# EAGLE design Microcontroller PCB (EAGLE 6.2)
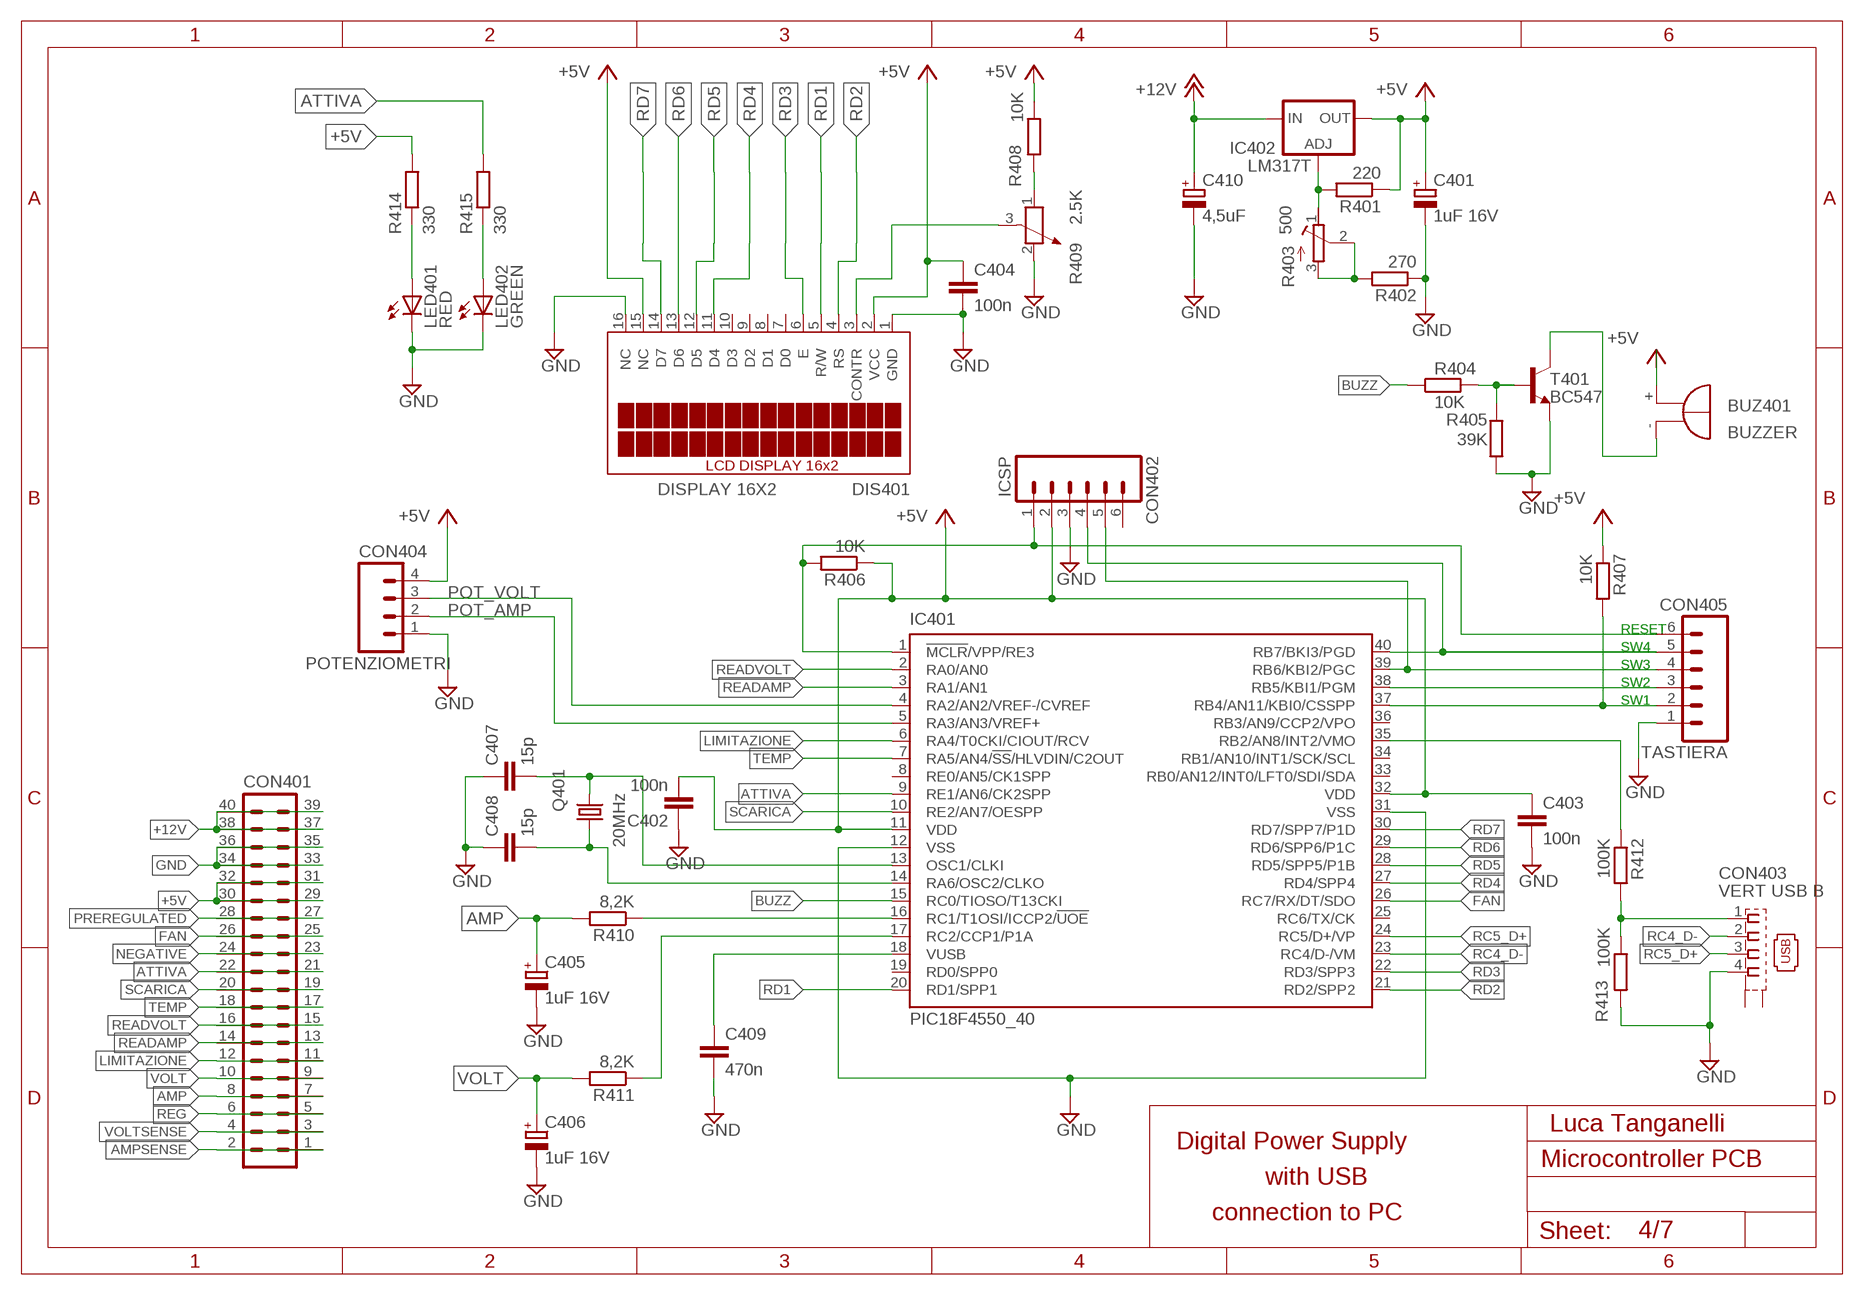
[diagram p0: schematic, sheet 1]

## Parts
BUZ401  BUZZER  F/HMB  [F/HMB]
C401  1uF 16V  CPOL-EUE2.5-5  [E2,5-5]
C402  100n  C-EU025-024X044  [C025-024X044]
C403  100n  C-EU025-024X044  [C025-024X044]
C404  100n  C-EU025-024X044  [C025-024X044]
C405  1uF 16V  CPOL-EUE2.5-5  [E2,5-5]
C406  1uF 16V  CPOL-EUE2.5-5  [E2,5-5]
C407  15p  C-EU025-024X044  [C025-024X044]
C408  15p  C-EU025-024X044  [C025-024X044]
C409  470n  C-EU050-024X044  [C050-024X044]
C410  4,5uF  CPOL-EUE2.5-5  [E2,5-5]
CON401  ML40  [ML40]
CON402  ICSP  MA06  [06PA]
CON403  VERT USB B  KUSBVX-BS1N  [KUSBVX-BS1N]
CON404  POTENZIOMETRI  MA04  [04PA]
CON405  TASTIERA  MA06  [06PA]
DIS401  DISPLAY 16X2  TUXGR_16X2_R2  [TUXGR_16X2_R2]
IC401  PIC18F4550_40  [DIL40]
IC402  LM317T  LM317TS  [317TS]
LED401  RED  LED3MM  [LED3MM]
LED402  GREEN  LED3MM  [LED3MM]
Q401  20MHz  CRYSTALHC49S  [HC49/S]
R401  220  R-EU_0207/10  [0207/10]
R402  270  R-EU_0207/10  [0207/10]
R403  500  R-TRIMMT93YA  [RTRIMT93YA]
R404  10K  R-EU_0207/15  [0207/15]
R405  39K  R-EU_0207/10  [0207/10]
R406  10K  R-EU_0207/22  [0207/22]
R407  10K  R-EU_0207/10  [0207/10]
R408  10K  R-EU_0207/10  [0207/10]
R409  2.5K  POTENTIOMETER_PT-10  [PT-10]
R410  8,2K  R-EU_0207/26  [0207/26]
R411  8,2K  R-EU_0207/26  [0207/26]
R412  100K  R-EU_0207/10  [0207/10]
R413  100K  R-EU_0207/10  [0207/10]
R414  330  R-EU_0207/10  [0207/10]
R415  330  R-EU_0207/22  [0207/22]
T401  BC547  BC547-NPN-TO92-CBE  [TO92-CBE]

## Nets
+5V: BUZ401.+ C401.+ C402.2 C403.1 C404.1 CON401.29 CON401.30 CON401.31 CON401.32 CON402.2 CON404.4 DIS401.2(VCC) DIS401.15(NC) IC401.11(VDD) IC401.32(VDD) IC402.2(OUT) R401.1 R406.1 R407.1 R408.1 R414.2
+12V: C410.+ CON401.37 CON401.38 CON401.39 CON401.40 IC402.3(IN)
AMP: C405.+ CON401.7 CON401.8 R410.2
AMPSENSE: CON401.1 CON401.2
ATTIVA: CON401.21 CON401.22 IC401.9(RE1/AN6/CK2SPP) R415.2
BUZZ: IC401.15(RC0/TIOSO/T13CKI) R404.1
FAN: CON401.25 CON401.26 IC401.26(RC7/RX/DT/SDO)
GND: C401.- C402.1 C403.2 C404.2 C405.- C406.- C407.1 C408.1 C409.2 C410.- CON401.33 CON401.34 CON401.35 CON401.36 CON402.3 CON403.4 CON404.1 CON405.1 DIS401.1(GND) DIS401.16(NC) IC401.12(VSS) IC401.31(VSS) LED401.K(C) LED402.K(C) R402.1 R405.1 R409.2 R413.2 T401.E
LIMITAZIONE: CON401.11 CON401.12 IC401.6(RA4/T0CKI/CIOUT/RCV)
N$1: CON405.3 IC401.38(RB5/KBI1/PGM)
N$2: CON405.2 IC401.37(RB4/AN11/KBI0/CSSPP) R407.2
N$7: IC401.35(RB2/AN8/INT2/VMO) R412.1
N$33: IC402.1(ADJ) R401.2 R403.1(A)
N$34: R402.2 R403.2(S) R403.3(E)
N$35: LED401.A R414.1
N$42: LED402.A R415.1
N$50: CON402.4 CON405.5 IC401.40(RB7/BKI3/PGD)
N$60: CON402.5 CON405.4 IC401.39(RB6/KBI2/PGC)
N$69: IC401.16(RC1/T1OSI/ICCP2/!UOE) R410.1
N$70: IC401.17(RC2/CCP1/P1A) R411.1
N$78: DIS401.3(CONTR) R409.3
N$82: CON403.1 R412.2 R413.1
N$83: C409.1 IC401.18(VUSB)
N$84: C408.2 IC401.14(RA6/OSC2/CLKO) Q401.1
N$85: C407.2 IC401.13(OSC1/CLKI) Q401.2
N$89: R408.2 R409.1
N$91: BUZ401.- T401.C
N$92: R404.2 R405.2 T401.B
NEGATIVE: CON401.23 CON401.24
POT_AMP: CON404.2 IC401.5(RA3/AN3/VREF+)
POT_VOLT: CON404.3 IC401.4(RA2/AN2/VREF-/CVREF)
PREREGULATED: CON401.27 CON401.28
RC4_D-: CON403.2 IC401.23(RC4/D-/VM)
RC5_D+: CON403.3 IC401.24(RC5/D+/VP)
RD1: DIS401.5(R/W) IC401.20(RD1/SPP1)
RD2: DIS401.4(RS) IC401.21(RD2/SPP2)
RD3: DIS401.6(E) IC401.22(RD3/SPP3)
RD4: DIS401.11(D4) IC401.27(RD4/SPP4)
RD5: DIS401.12(D5) IC401.28(RD5/SPP5/P1B)
RD6: DIS401.13(D6) IC401.29(RD6/SPP6/P1C)
RD7: DIS401.14(D7) IC401.30(RD7/SPP7/P1D)
READAMP: CON401.13 CON401.14 IC401.3(RA1/AN1)
READVOLT: CON401.15 CON401.16 IC401.2(RA0/AN0)
REG: CON401.5 CON401.6
RESET: CON402.1 CON405.6 IC401.1(!MCLR!/VPP/RE3) R406.2
SCARICA: CON401.19 CON401.20 IC401.10(RE2/AN7/OESPP)
TEMP: CON401.17 CON401.18 IC401.7(RA5/AN4/!SS!/HLVDIN/C2OUT)
VOLT: C406.+ CON401.9 CON401.10 R411.2
VOLTSENSE: CON401.3 CON401.4
Unconnected: CON402.6 CON403.M1(S1) CON403.M2(S2) DIS401.7(D0) DIS401.8(D1) DIS401.9(D2) DIS401.10(D3) IC401.8(RE0/AN5/CK1SPP) IC401.19(RD0/SPP0) IC401.25(RC6/TX/CK) IC401.33(RB0/AN12/INT0/LFT0/SDI/SDA) IC401.34(RB1/AN10/INT1/SCK/SCL) IC401.36(RB3/AN9/CCP2/VPO)

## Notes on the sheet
- RESET
- SW4
- SW3
- SW2
- SW1
- Luca Tanganelli
- Digital Power Supply
- with USB
- connection to PC
- 4/7

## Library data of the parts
BUZ401 = buzzer:F/HMB: BUZZER; OC_FARNELL: unknown; OC_NEWARK: unknown
C401 C405 C406 C410 = #-rcl:CPOL-EU: POLARIZED CAPACITOR, European symbol
C402-C404 C407-C409 = #-rcl:C-EU: CAPACITOR, European symbol
CON401 = #-con-ml:ML40: HARTING; OC_FARNELL: unknown; OC_NEWARK: unknown
CON402 CON405 = #-con-amp-quick:MA06: AMP QUICK CONNECTOR; OC_FARNELL: unknown; OC_NEWARK: unknown
CON403 = #-con-kycon:KUSBVX-BS1N: USB B-type Receptacle Vertical, 4 Position, Through Hole Source: Sibalco Kycon KUSBVX-BS1N-xxx.pdf
CON404 = #-con-amp-quick:MA04: AMP QUICK CONNECTOR; OC_FARNELL: unknown; OC_NEWARK: unknown
DIS401 = #-display-lcd:TUXGR_16X2_R2: Tuxgraphics LCD display 16x2 characters reflective, without background light Source: tuxgr_12x2_r2.pdf; OC_FARNELL: unknown; OC_NEWARK: unknown
IC401 = #-microchip:PIC18F4*_40: USB Microcontrollers with nanoWatt Technology High-Performance, Enhanced Flash, 28/40/44-Pin, Source: http://ww1.microchip.com/downloads/en/devicedoc/39632c.pdf; MF: MICROCHIP; MPN: PIC18F4550-I/P; OC_FARNELL: 9321357; OC_NEWARK: 74K8623
IC402 = #-v-reg:LM317TS: VOLTAGE REGULATOR
LED401 LED402 = #-led:LED: LED
Q401 = #-crystal:CRYSTAL: CRYSTAL; OC_FARNELL: 1667008; OC_NEWARK: unknown
R401 R402 R404-R408 R410-R415 = #-rcl:R-EU_: RESISTOR, European symbol
R403 = #-rcl:R-TRIMM: Trimm resistor
R409 = #-rcl:POTENTIOMETER_: Potentiometer
T401 = #-transistor:*-NPN-: NPN Transistror BF959 corrected 2008.03.06

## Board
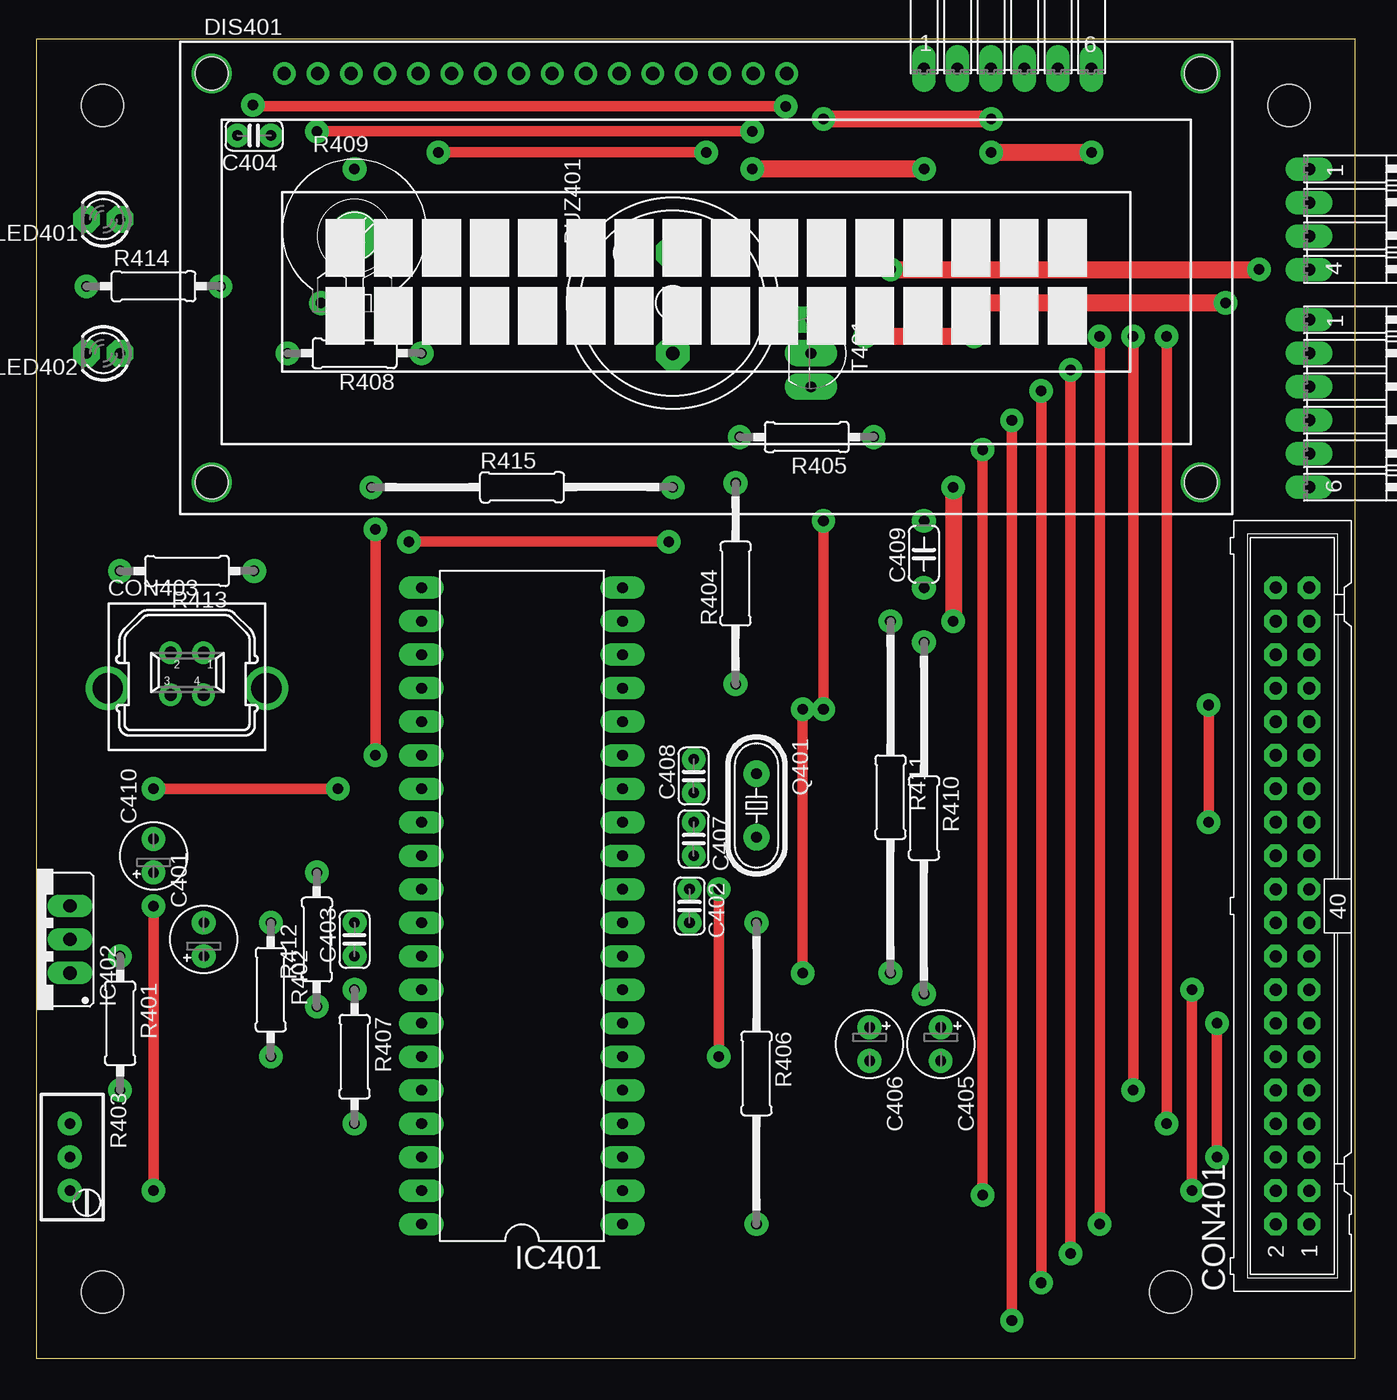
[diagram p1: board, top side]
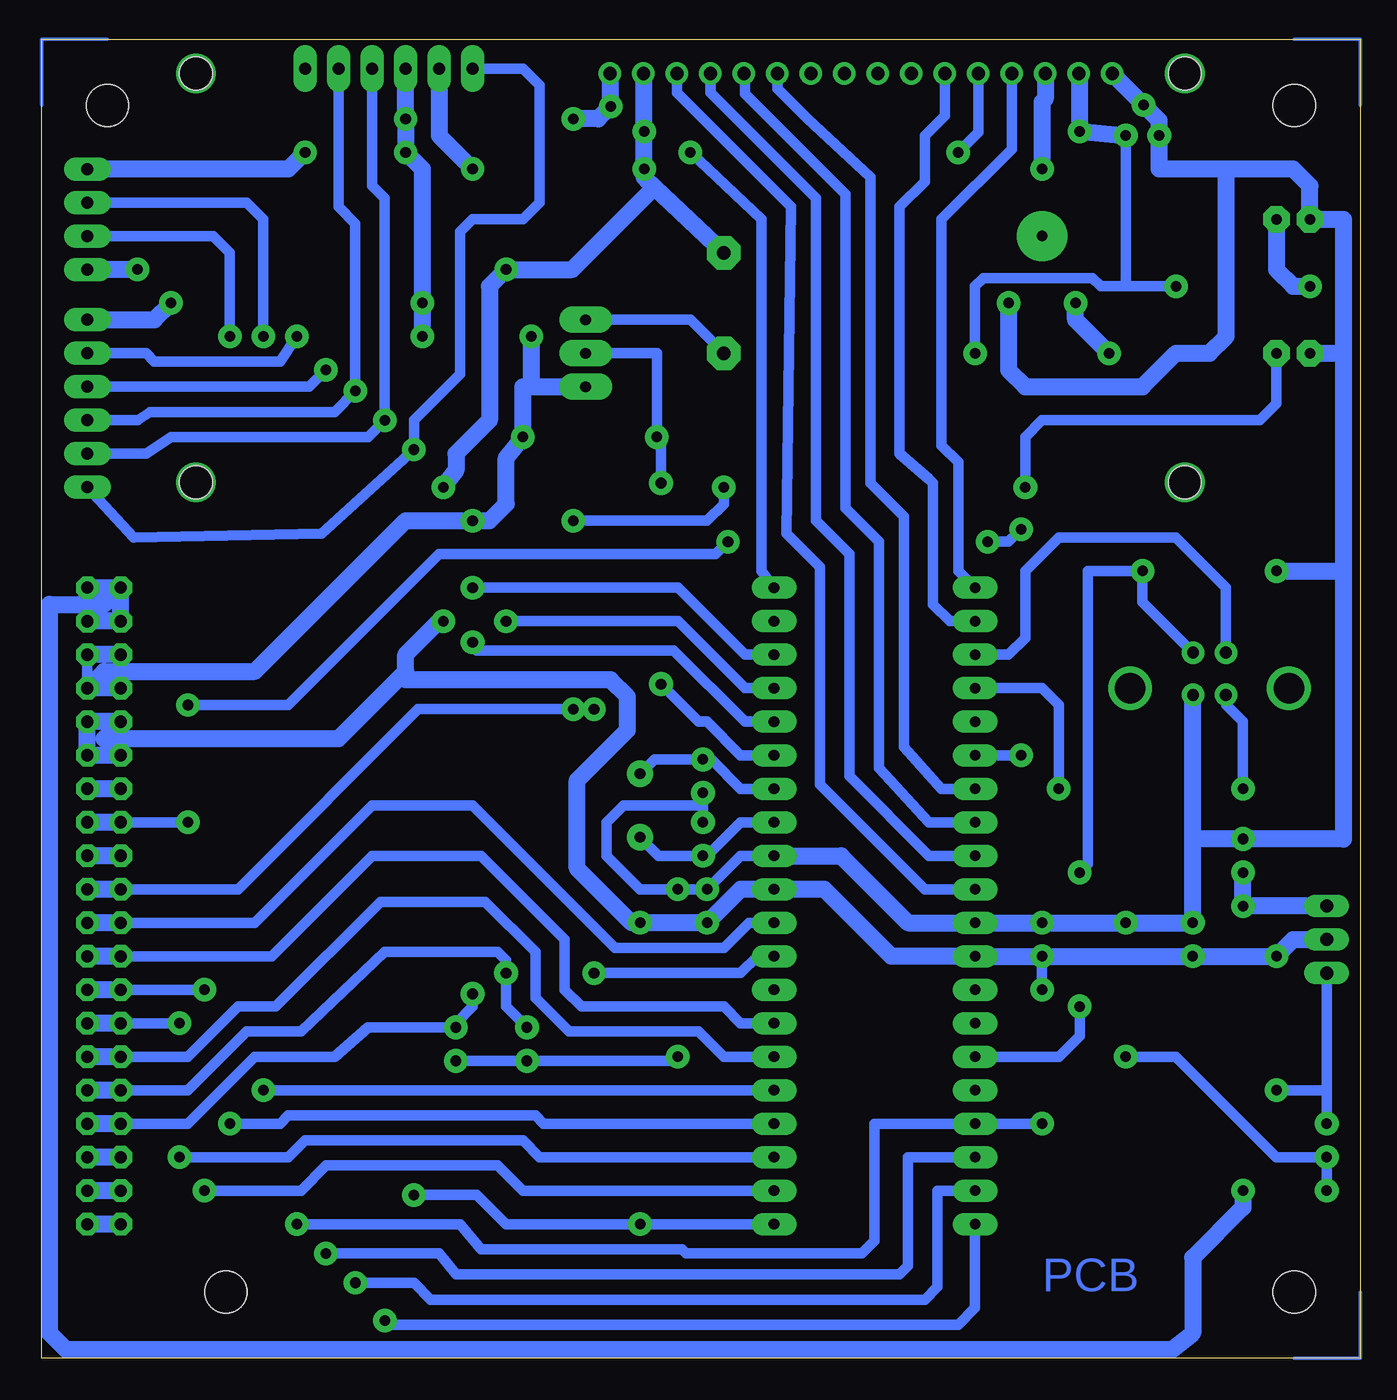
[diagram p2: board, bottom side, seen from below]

Size 100 x 100 mm. Coordinates in mm from the lower left corner, seen from the top.
Outline: 0,0 100,0 100,100 0,100 0,0
Copper layers (1*16): Top 0.035mm / dielectric 1.5mm / Bottom 0.035mm
Design rules: minimum track width 10mil, minimum drill 24mil, track to track 8mil, track to pad 8mil, pad to pad 8mil, via to via 8mil, smd to smd 8mil, copper to edge 40mil, drill to drill 8mil, minimum pad ring 10mil, minimum via ring 8mil, stop-mask expansion 4mil, vias tented up to drill 0mil, thermal gap 10mil
Holes 3.2 mm at 5,95 95,95 86,5 5,5

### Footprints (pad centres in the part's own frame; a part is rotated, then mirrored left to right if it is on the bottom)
F/HMB = drill 1.016 pad 2.54 octagon: + 3.81,0; - -3.81,0
E2,5-5 = drill 0.8 pad 1.8: + -1.27,0; - 1.27,0
C025-024X044 = drill 0.8 pad 1.8: 1 -1.27,0; 2 1.27,0
C050-024X044 = drill 0.8 pad 1.8: 1 -2.54,0; 2 2.54,0
ML40 = drill 0.914 pad 1.7 octagon: 1 -24.13,-1.27; 2 -24.13,1.27; 3 -21.59,-1.27; 4 -21.59,1.27; 5 -19.05,-1.27; 6 -19.05,1.27; 7 -16.51,-1.27; 8 -16.51,1.27; 9 -13.97,-1.27; 10 -13.97,1.27; 11 -11.43,-1.27; 12 -11.43,1.27; 13 -8.89,-1.27; 14 -8.89,1.27; 15 -6.35,-1.27; 16 -6.35,1.27; 17 -3.81,-1.27; 18 -3.81,1.27; 19 -1.27,-1.27; 20 -1.27,1.27; 21 1.27,-1.27; 22 1.27,1.27; 23 3.81,-1.27; 24 3.81,1.27; 25 6.35,-1.27; 26 6.35,1.27; 27 8.89,-1.27; 28 8.89,1.27; 29 11.43,-1.27; 30 11.43,1.27; 31 13.97,-1.27; 32 13.97,1.27; 33 16.51,-1.27; 34 16.51,1.27; 35 19.05,-1.27; 36 19.05,1.27; 37 21.59,-1.27; 38 21.59,1.27; 39 24.13,-1.27; 40 24.13,1.27
06PA = drill 0.914 pad 1.8 long: 1 -6.35,0; 2 -3.81,0; 3 -1.27,0; 4 1.27,0; 5 3.81,0; 6 6.35,0
KUSBVX-BS1N = drill 0.9 pad 1.7: 1 1.25,2.7; 2 -1.25,2.7; 3 -1.25,-0.5; 4 1.25,-0.5 | drill 2.3 pad 1.7: M1 -6.02,0; M2 6.02,0
04PA = drill 0.914 pad 1.8 long: 1 -3.81,0; 2 -1.27,0; 3 1.27,0; 4 3.81,0
TUXGR_16X2_R2 = drill 1 pad 1.7: 1 -32,15.5; 2 -29.46,15.5; 3 -26.92,15.5; 4 -24.38,15.5; 5 -21.84,15.5; 6 -19.3,15.5; 7 -16.76,15.5; 8 -14.22,15.5; 9 -11.68,15.5; 10 -9.14,15.5; 11 -6.6,15.5; 12 -4.06,15.5; 13 -1.52,15.5; 14 1.02,15.5; 15 3.56,15.5; 16 6.1,15.5 | hole 2.5: -37.5,-15.5; 37.5,-15.5; -37.5,15.5; 37.5,15.5
DIL40 = drill 0.813 pad 1.7 long: 1 -24.13,-7.62; 2 -21.59,-7.62; 3 -19.05,-7.62; 4 -16.51,-7.62; 5 -13.97,-7.62; 6 -11.43,-7.62; 7 -8.89,-7.62; 8 -6.35,-7.62; 9 -3.81,-7.62; 10 -1.27,-7.62; 11 1.27,-7.62; 12 3.81,-7.62; 13 6.35,-7.62; 14 8.89,-7.62; 15 11.43,-7.62; 16 13.97,-7.62; 17 16.51,-7.62; 18 19.05,-7.62; 19 21.59,-7.62; 20 24.13,-7.62; 21 24.13,7.62; 22 21.59,7.62; 23 19.05,7.62; 24 16.51,7.62; 25 13.97,7.62; 26 11.43,7.62; 27 8.89,7.62; 28 6.35,7.62; 29 3.81,7.62; 30 1.27,7.62; 31 -1.27,7.62; 32 -3.81,7.62; 33 -6.35,7.62; 34 -8.89,7.62; 35 -11.43,7.62; 36 -13.97,7.62; 37 -16.51,7.62; 38 -19.05,7.62; 39 -21.59,7.62; 40 -24.13,7.62
317TS = drill 1.016 pad 1.7 long: 1 -2.54,-2.54; 2 0,-2.54; 3 2.54,-2.54
LED3MM = drill 0.813 pad 2 octagon: A -1.27,0; K 1.27,0
HC49/S = drill 0.813 pad 2: 1 -2.413,0; 2 2.413,0
0207/10 = drill 0.8 pad 1.8: 1 -5.08,0; 2 5.08,0
RTRIMT93YA = drill 0.8 pad 1.8: 1 0,-2.54; 2 0,0; 3 0,2.54
0207/15 = drill 0.8 pad 1.8: 1 -7.62,0; 2 7.62,0
0207/22 = drill 0.8 pad 1.8: 1 -11.43,0; 2 11.43,0
PT-10 = drill 0.8 pad 1.8: 1 -2.54,-5.08; 2 2.54,-5.08; 3 0,5.08
0207/26 = drill 0.8 pad 1.8: 1 -13.335,0; 2 13.335,0
TO92-CBE = drill 0.813 pad 2 long: B 0,0; C -2.54,0; E 2.54,0

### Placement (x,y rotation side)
BUZ401  48.26,80.01 90 top
C401  12.7,31.75 90 top
C402  49.53,34.29 270 top
C403  24.13,31.75 90 top
C404  16.51,92.71 180 top
C405  68.58,23.81 270 top
C406  63.18,23.81 270 top
C407  49.85,39.37 270 top
C408  49.85,44.13 90 top
C409  67.31,60.96 90 top
C410  8.89,38.1 90 top
CON401  95.25,34.29 90 top
CON402  73.66,97.79 0 top
CON403  11.43,50.8 0 top
CON404  96.52,86.36 270 top
CON405  96.52,72.39 270 top
DIS401  50.8,81.92 0 top
IC401  36.83,34.29 90 top
IC402  0,31.75 90 top
LED401  5.08,86.36 180 top
LED402  5.08,76.2 180 top
Q401  54.61,41.91 270 top
R401  6.35,25.4 270 top
R402  17.78,27.94 270 top
R403  2.54,15.24 180 top
R404  53.02,58.74 90 top
R405  58.42,69.85 180 top
R406  54.61,21.59 270 top
R407  24.13,22.86 270 top
R408  24.13,76.2 180 top
R409  24.13,85.09 0 top
R410  67.31,40.96 270 top
R411  64.77,42.55 270 top
R412  21.27,31.75 90 top
R413  11.43,59.69 180 top
R414  8.89,81.28 0 top
R415  36.83,66.04 0 top
T401  58.74,76.2 270 top

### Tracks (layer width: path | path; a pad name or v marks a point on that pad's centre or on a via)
+5V  (via drill 0.8 pad 1.78)
  Top 0.813: v54.29,93.03 v21.27,93.03
  Top 1.27: v64.77,82.55 v92.71,82.55 | v67.31,90.17 v54.29,90.17 | v69.53,66.04 v69.53,55.88
  Bottom 0.813: R407.1 C403.1 | R408.1 29.21,81.28 28.57,81.92 20.32,81.92 19.68,81.28 17.78,81.28 | 17.78,81.28 R414.2 | C404.1 17.78,81.28 | 72.39,51.44 72.39,52.07
  Bottom 1.27: IC402.2 5.08,31.75 R401.1 C401.+ C403.1 IC401.32 35.56,30.48 40.64,35.56 IC401.11 46.99,35.56 C402.2 R406.1 55.24,33.02 59.37,37.15 59.37,43.81 55.56,47.62 55.56,50.16 56.83,51.44 72.39,51.44 | BUZ401.+ 53.51,88.79 | 53.51,88.79 54.14,89.39 | 54.14,89.39 54.29,89.53 v54.29,90.17 | v54.29,90.17 v54.29,93.03 54.29,97.35 DIS401.15 | DIS401.2 21.27,97.35 v21.27,93.03 C404.1 | v92.71,82.55 CON404.4 | CON402.2 69.85,92.71 v67.31,90.17 | v54.29,90.17 54.29,89.54 54.14,89.39 | 53.51,88.79 59.75,82.55 v64.77,82.55 66.04,81.28 66.04,71.12 68.58,68.58 68.58,67.31 v69.53,66.04 | CON401.30 CON401.29 CON401.31 CON401.32 95.25,46.99 77.47,46.99 72.39,52.07 72.39,53.34 69.85,55.88 v69.53,55.88
+12V  (via drill 0.8 pad 1.78)
  Top 0.813: v8.89,34.29 v8.89,12.7
  Bottom 1.27: IC402.3 v8.89,34.29 C410.+ | CON401.40 CON401.39 CON401.37 CON401.38 CON401.40 | CON401.40 95.25,57.15 99.38,57.15 99.38,1.91 98.11,0.64 14.29,0.64 12.7,1.91 12.7,7.62 8.89,11.43 v8.89,12.7
AMP
  Bottom 0.813: R410.2 67.31,26.99 67.31,26.67 68.58,25.4 C405.+ 75.25,25.08 77.79,22.86 83.82,22.86 88.9,17.78 CON401.8
  Bottom 1.27: CON401.8 CON401.7
AMPSENSE
  Bottom 1.27: CON401.2 CON401.1
ATTIVA  (via drill 0.8 pad 1.78)
  Top 0.813: v58.1,29.21 v58.1,49.21 | v59.69,63.5 v59.69,49.21
  Bottom 0.813: IC401.9 45.72,30.48 46.99,29.21 v58.1,29.21 | CON401.22 85.09,35.56 71.44,49.21 v59.69,49.21 v58.1,49.21 | R415.2 48.26,64.77 49.53,63.5 v59.69,63.5
  Bottom 1.27: CON401.22 CON401.21
BUZZ
  Bottom 0.813: IC401.15 46.99,45.72 49.53,48.26 50.16,48.26 R404.1
FAN  (via drill 0.8 pad 1.78)
  Top 0.813: v28.26,61.91 v47.94,61.91 | v88.9,49.53 v88.9,40.64 | v25.72,62.87 v25.72,45.72
  Bottom 0.813: v47.94,61.91 48.9,60.96 69.85,60.96 81.28,49.53 v88.9,49.53 | v88.9,40.64 CON401.26 | v28.26,61.91 26.67,61.91 v25.72,62.87 | v25.72,45.72 IC401.26
  Bottom 1.27: CON401.26 CON401.25
GND  (via drill 0.8 pad 1.78)
  Top 0.813: v56.83,94.93 16.51,94.93 | v51.75,22.86 v51.75,35.56
  Top 1.27: 16.51,94.93 v16.41,95.03 | v59.69,93.98 v72.39,93.98 | v72.39,91.44 v80.01,91.44 | v71.12,77.47 v62.87,77.47 | v90.17,80.01 v71.12,80.01
  Bottom 0.813: C407.1 49.85,41.91 | 49.85,41.91 C408.1 | IC401.12 46.99,38.1 C402.1 v51.75,35.56 54.61,35.56 57.15,38.1 57.15,40.64 55.88,41.91 49.85,41.91 | 12.7,50.28 CON403.4 | CON401.35 CON401.33 | v51.75,22.86 52.39,22.54 C406.- C405.-
  Bottom 1.27: IC401.12 39.37,38.1 34.29,33.02 IC401.31 C403.2 R402.1 C401.- 12.7,39.37 | 12.7,39.37 12.7,50.28 | R413.2 1.27,59.69 | 1.27,59.69 1.27,39.37 C410.- 12.7,39.37 | LED402.K 1.27,76.2 | 1.27,76.2 1.27,59.69 | 1.27,76.2 1.27,86.36 LED401.K 3.81,88.9 5.08,90.17 10.16,90.17 | 10.16,90.17 15.24,90.17 C404.2 15.24,93.86 v16.41,95.03 DIS401.1 | R409.2 26.67,74.93 25.4,73.66 16.51,73.66 13.97,76.2 11.43,76.2 10.16,77.47 10.16,90.17 | DIS401.16 56.9,95 v56.83,94.93 57.78,93.98 v59.69,93.98 | CON402.3 v72.39,93.98 v72.39,91.44 71.12,90.17 v71.12,80.01 v71.12,77.47 | v80.01,91.44 81.28,90.17 CON404.1 | v62.87,77.47 62.87,73.66 T401.E 63.5,73.66 R405.1 64.77,68.26 64.77,64.77 66.04,63.5 C409.2 72.39,63.5 83.82,52.07 95.25,52.07 CON401.33 CON401.34 | CON405.1 91.44,78.74 v90.17,80.01 | CON401.36 CON401.35
LIMITAZIONE
  Bottom 0.813: CON401.12 88.9,22.86 85.09,26.67 82.23,26.67 74.3,34.61 66.36,34.61 62.55,30.8 62.55,27.3 60.01,24.77 50.16,24.77 48.26,22.86 IC401.6
  Bottom 1.27: CON401.12 CON401.11
N$1  (via drill 0.8 pad 1.78)
  Top 0.813: v78.42,7.94 v78.42,74.93
  Bottom 0.813: IC401.38 34.29,15.24 34.29,6.99 34.92,6.35 68.58,6.35 69.85,7.94 v78.42,7.94 | v78.42,74.93 79.69,73.66 CON405.3
N$2  (via drill 0.8 pad 1.78)
  Top 0.813: v80.64,10.16 v80.64,77.47
  Bottom 0.813: R407.2 IC401.37 36.83,17.78 36.83,8.89 37.78,7.94 51.12,7.94 51.44,8.26 66.67,8.26 68.26,10.16 v80.64,10.16 | v80.64,77.47 81.92,75.56 91.44,75.56 92.08,76.2 CON405.2
N$3  (via drill 0.8 pad 3.81)
  other vias: 24.13,85.09
N$4
  Bottom 0.254: 0,95 0,100 5,100
N$5
  Bottom 0.254: 95,100 100,100 100,95
N$6
  Bottom 0.254: 0,5 0,0 5,0
N$7
  Bottom 0.813: IC401.35 22.86,22.86 21.27,24.45 R412.1
N$33
  Bottom 0.813: IC402.1 2.54,20.32 | 2.54,20.32 R403.1 | R401.2 2.54,20.32
N$34
  Bottom 0.813: R403.3 R403.2 6.35,15.24 13.97,22.86 R402.2
N$35
  Bottom 1.27: LED401.A 6.35,82.55 5.08,81.28 R414.1
N$42
  Bottom 0.813: LED402.A 6.35,72.39 7.62,71.12 24.13,71.12 25.4,69.85 R415.1
N$50  (via drill 0.8 pad 1.78)
  Top 0.813: v73.98,2.86 v73.98,71.12
  Bottom 0.813: IC401.40 29.21,3.81 30.48,2.54 73.66,2.54 v73.98,2.86 | CON402.4 74.93,88.9 73.98,87.95 v73.98,71.12 75.25,69.85 90.17,69.85 92.08,68.58 CON405.5
N$60  (via drill 0.8 pad 1.78)
  Top 0.813: v76.2,5.71 v76.2,73.34
  Bottom 0.813: IC401.39 32.07,12.7 32.07,5.4 33.02,4.45 70.48,4.45 71.75,5.71 v76.2,5.71 | CON402.5 77.47,87.31 76.2,86.04 v76.2,73.34 77.79,71.75 91.76,71.75 92.71,71.12 CON405.4
N$69
  Bottom 0.813: IC401.16 46.67,48.26 52.07,53.66 66.99,53.66 R410.1
N$70
  Bottom 0.813: IC401.17 46.67,50.8 51.75,55.88 R411.1
N$78
  Bottom 1.27: DIS401.3 23.88,95.5 24.13,95.25 R409.3
N$82
  Bottom 0.813: CON403.1 16.51,57.33 R413.1 20.64,59.69 20.64,37.47 R412.2
N$83
  Bottom 0.813: IC401.18 46.67,53.34 51.75,58.42 C409.1
N$84
  Bottom 0.813: Q401.1 53.53,45.4 C408.2 49.21,45.4 46.99,43.18 IC401.14
N$85
  Bottom 0.813: Q401.2 53.21,38.1 C407.2 49.53,38.1 46.99,40.64 IC401.13
N$89
  Bottom 1.27: R408.2 21.59,78.74 R409.1
N$91
  Bottom 0.813: BUZ401.- 50.8,78.74 T401.C
N$92
  Bottom 0.813: T401.B 53.34,76.2 R405.2 53.02,69.53 R404.2
NEGATIVE
  Bottom 1.27: CON401.24 CON401.23
POT_AMP  (via drill 0.8 pad 1.78)
  Top 0.813: v83.19,77.47 v83.19,20.32
  Bottom 0.813: v83.19,77.47 83.19,86.36 84.45,87.63 CON404.2 | IC401.5 v83.19,20.32
POT_VOLT  (via drill 0.8 pad 1.78)
  Top 0.813: v85.72,77.47 v85.72,17.78
  Bottom 0.813: v85.72,77.47 85.72,83.82 87,85.09 CON404.3 | IC401.4 61.91,17.78 62.55,18.41 81.28,18.41 81.92,17.78 v85.72,17.78
PREREGULATED
  Bottom 1.27: CON401.28 CON401.27
RC4_D-
  Bottom 0.813: CON403.2 10.18,58.44 13.97,62.23 22.86,62.23 25.4,59.69 25.4,54.61 26.67,53.34 IC401.23
RC5_D+  (via drill 0.8 pad 1.78)
  Top 0.813: v22.86,43.18 v8.89,43.18
  Bottom 0.813: IC401.24 24.13,50.8 22.86,49.53 v22.86,43.18 | v8.89,43.18 8.89,48.26 10.16,49.53 10.16,50.28 CON403.3
RD1  (via drill 0.8 pad 1.78)
  Top 0.813: v30.48,91.44 v50.8,91.44
  Bottom 0.813: DIS401.5 28.96,92.96 v30.48,91.44 | v50.8,91.44 45.4,86.36 45.4,59.69 IC401.20
RD2
  Bottom 0.813: DIS401.4 26.42,91.69 31.75,86.36 31.75,69.22 30.48,67.94 30.48,59.69 IC401.21
RD3
  Bottom 0.813: DIS401.6 31.5,94.23 33.02,92.71 33.02,89.22 34.92,87.31 34.92,68.58 32.7,66.67 32.38,66.36 32.38,57.15 31.11,55.88 IC401.22
RD4
  Bottom 0.813: DIS401.11 44.2,96.27 41.91,93.98 37.15,89.53 37.15,66.36 34.61,63.82 34.61,46.35 31.75,43.18 IC401.27
RD5
  Bottom 0.813: IC401.28 32.7,40.64 36.51,44.77 36.51,61.91 39.05,64.45 39.05,88.27 46.67,95.89 46.67,97.35 DIS401.12
RD6
  Bottom 0.813: DIS401.13 49.28,95.95 41.27,87.95 41.27,63.5 38.73,60.96 38.73,44.13 32.7,38.1 IC401.29
RD7
  Bottom 0.813: DIS401.14 51.82,95.95 43.18,87.31 43.5,62.55 40.96,60.01 40.96,43.5 33.02,35.56 IC401.30
READAMP  (via drill 0.8 pad 1.78)
  Top 0.813: v89.53,25.4 v89.53,15.24
  Bottom 0.813: CON401.14 v89.53,25.4 | v89.53,15.24 81.28,15.24 80.01,16.51 63.5,16.51 62.23,15.24 IC401.3
  Bottom 1.27: CON401.14 CON401.13
READVOLT  (via drill 0.8 pad 1.78)
  Top 0.813: v87.63,12.7 v87.63,27.94
  Bottom 0.813: IC401.2 63.5,12.7 65.41,14.61 78.42,14.61 80.33,12.7 v87.63,12.7 | v87.63,27.94 CON401.16
  Bottom 1.27: CON401.16 CON401.15
REG
  Bottom 1.27: CON401.6 CON401.5
RESET  (via drill 0.8 pad 1.78)
  Top 0.813: v71.75,12.38 v71.75,68.9
  Bottom 0.813: CON405.6 93.03,62.23 78.74,62.55 v71.75,68.9 71.75,71.12 68.26,74.61 68.26,85.41 67.31,86.36 63.5,86.36 62.23,87.63 62.23,96.52 63.5,97.79 CON402.1 | IC401.1 R406.2 64.77,10.16 66.99,12.38 v71.75,12.38
S$1  (via drill 0.6 pad 3)
  other vias: 5,5
S$2  (via drill 0.6 pad 3)
  other vias: 5,95
S$3  (via drill 0.6 pad 3)
  other vias: 95,95
S$4  (via drill 0.6 pad 3)
  other vias: 86,5
S$5  (via drill 0.6 pad 3)
  other vias: 88.3,66.4
S$6  (via drill 0.6 pad 3)
  other vias: 88.3,97.41
S$7  (via drill 0.6 pad 3)
  other vias: 13.3,97.41
S$8  (via drill 0.6 pad 3)
  other vias: 13.3,66.4
SCARICA
  Bottom 0.813: IC401.10 46.35,33.02 48.26,31.11 56.52,31.11 67.31,41.91 74.93,41.91 83.82,33.02 CON401.20
  Bottom 1.27: CON401.20 CON401.19
TEMP
  Bottom 0.813: CON401.18 82.55,30.48 74.93,38.1 66.67,38.1 60.33,31.75 60.33,27.94 59.05,26.67 48.26,26.67 46.99,25.4 IC401.7
  Bottom 1.27: CON401.18 CON401.17
VOLT
  Bottom 0.813: C406.+ 64.77,26.67 R411.2 64.77,30.16 65.41,30.8 73.98,30.8 80.33,24.77 84.45,24.77 88.9,20.32 CON401.10
  Bottom 1.27: CON401.10 CON401.9
VOLTSENSE
  Bottom 1.27: CON401.4 CON401.3

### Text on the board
Bottom: PCB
